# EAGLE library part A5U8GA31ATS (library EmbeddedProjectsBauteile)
Zentel 1G x 8bit NAND Flash Memory
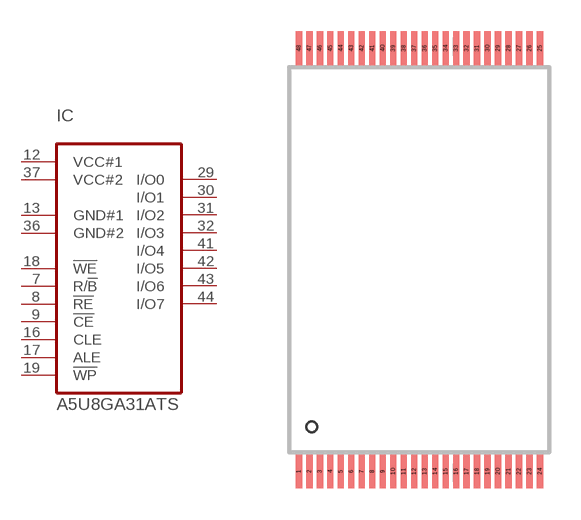
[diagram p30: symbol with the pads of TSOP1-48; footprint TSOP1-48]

Designator prefix IC

## A5U8GA31ATS  [TSOP1-48]
7  R/!B  in
8  !RE  in
9  !CE  in
12  VCC#1  pwr
13  GND#1  pwr
16  CLE  in
17  ALE  in
18  !WE  in
19  !WP  in
29  I/O0
30  I/O1
31  I/O2
32  I/O3
36  GND#2  pwr
37  VCC#2  pwr
41  I/O4
42  I/O5
43  I/O6
44  I/O7

## Footprint TSOP1-48 (pad centres in mm)
smd 0.3 x 1.6: 1 -5.75,-10.1; 2 -5.25,-10.1; 3 -4.75,-10.1; 4 -4.25,-10.1; 5 -3.75,-10.1; 6 -3.25,-10.1; 7 -2.75,-10.1; 8 -2.25,-10.1; 9 -1.75,-10.1; 10 -1.25,-10.1; 11 -0.75,-10.1; 12 -0.25,-10.1; 13 0.25,-10.1; 14 0.75,-10.1; 15 1.25,-10.1; 16 1.75,-10.1; 17 2.25,-10.1; 18 2.75,-10.1; 19 3.25,-10.1; 20 3.75,-10.1; 21 4.25,-10.1; 22 4.75,-10.1; 23 5.25,-10.1; 24 5.75,-10.1; 25 5.75,10.1; 26 5.25,10.1; 27 4.75,10.1; 28 4.25,10.1; 29 3.75,10.1; 30 3.25,10.1; 31 2.75,10.1; 32 2.25,10.1; 33 1.75,10.1; 34 1.25,10.1; 35 0.75,10.1; 36 0.25,10.1; 37 -0.25,10.1; 38 -0.75,10.1; 39 -1.25,10.1; 40 -1.75,10.1; 41 -2.25,10.1; 42 -2.75,10.1; 43 -3.25,10.1; 44 -3.75,10.1; 45 -4.25,10.1; 46 -4.75,10.1; 47 -5.25,10.1; 48 -5.75,10.1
